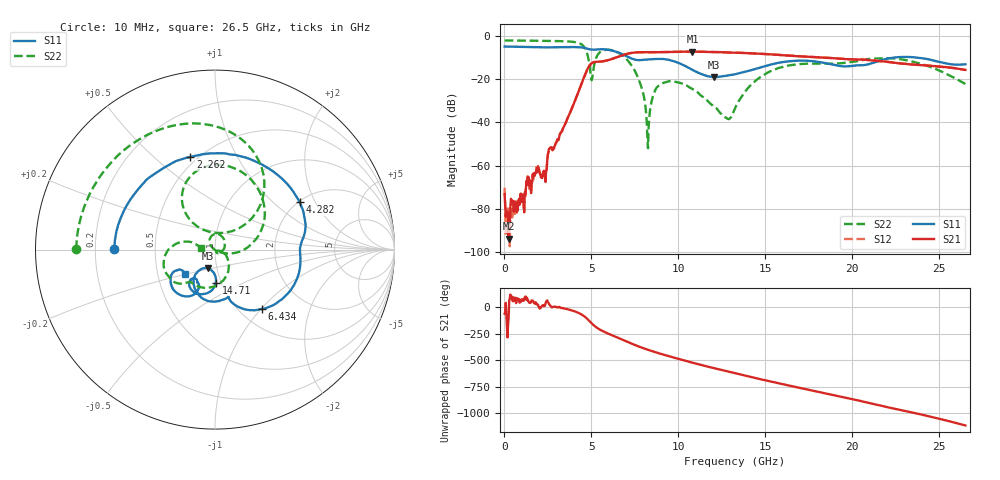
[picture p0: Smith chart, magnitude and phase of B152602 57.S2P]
!  2-Port S-parameters saved by WinCal
! VAR MeasName=S-Parameters (CALIBRATED_DATA) read from VNA (N5242A)
! VAR MeasDate=2016-1-5 16:34:05
! VAR NAME=B152602 57
! VAR FILENAME=B152602 57.S2P
! VAR DATE=2016-1-5 16:34:05
! VAR PHYS_PORTS=1,2
# Hz S DB R 50
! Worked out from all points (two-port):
!   801 points, 10 MHz to 26.5 GHz, reference 50 ohm
!   highest |S21| = -7.40 dB at 10.8 GHz (marker M1); lowest = -93.7 dB at 241.8 MHz (marker M2)
!   |S21| within 3 dB of the highest: 6.307 GHz to 18.89 GHz (12.59 GHz wide, 99.9 % of centre)
!   lowest |S11| = -19.2 dB at 12.03 GHz (marker M3), VSWR 1.25, Z = 45.3 - j9.46 ohm
!   |S11| at or under -10 dB: 7.15 GHz to 22.55 GHz (15.4 GHz wide, 104 % of centre); 23.51 GHz to end of sweep
!   |S22| runs from -52.0 to -2.2 dB; largest |S21 - S12| = 0.0034
!   S11 on the Smith chart (normalised r, x): 10 MHz: 0.28, +0.00; 2.262 GHz: 0.46, +0.66; 4.282 GHz: 2.03, +1.51; 6.434 GHz: 1.25, -1.00; 14.71 GHz: 0.94, -0.36; 26.5 GHz: 0.69, -0.20
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1e7  -5.03 179.6  -73.10 -60.2  -70.19 12.5  -2.25 179.8
2.417875e8  -5.05 171.7  -93.71 -104.0  -81.28 -30.7  -2.25 176.3
1.0696e9  -5.27 144.4  -74.64 61.5  -73.65 67.6  -2.30 163.4
1.831188e9  -5.40 119.5  -62.00 28.0  -60.82 25.9  -2.37 151.1
2.26165e9  -5.44 104.9  -62.34 10.6  -63.13 11.6  -2.42 143.6
2.592775e9  -5.41 93.8  -52.15 23.8  -52.31 25.7  -2.45 137.4
4.281512e9  -5.34 29.2  -25.38 -54.6  -25.39 -54.5  -3.45 85.5
4.447075e9  -5.46 21.8  -21.86 -69.3  -21.87 -69.1  -4.13 74.5
5.009988e9  -6.47 1.7  -12.78 -150.2  -12.79 -150.1  -20.63 83.3
5.506675e9  -6.28 -14.2  -12.00 148.1  -12.01 148.3  -7.54 110.9
6.433825e9  -7.54 -51.9  -10.04 79.5  -10.02 79.6  -7.41 58.4
7.625875e9  -11.28 -73.9  -7.73 -3.1  -7.71 -3.0  -18.45 -8.0
8.2219e9  -11.01 -79.0  -7.69 -38.9  -7.66 -38.8  -47.95 -58.3
8.851038e9  -10.77 -91.1  -7.66 -71.5  -7.62 -71.5  -23.20 112.9
1.080468e10  -15.81 -128.2  -7.40 -161.3  -7.38 -161.4  -24.60 22.1
1.202984e10  -19.15 -110.7  -7.58 147.4  -7.58 147.3  -32.63 -56.6
1.285765e10  -18.37 -97.4  -7.78 114.0  -7.77 114.1  -38.49 -44.3
1.3255e10  -17.83 -93.0  -7.88 98.7  -7.87 98.7  -33.55 -15.9
1.471195e10  -14.71 -88.6  -8.39 43.1  -8.35 43.1  -19.16 -45.3
1.769208e10  -11.76 -121.6  -9.87 -64.0  -9.83 -63.9  -12.93 -115.6
2.209604e10  -10.49 -119.3  -12.23 136.7  -12.16 136.4  -10.40 -159.6
2.65e10  -13.22 -141.0  -15.83 -32.6  -15.83 -32.7  -22.36 172.4
